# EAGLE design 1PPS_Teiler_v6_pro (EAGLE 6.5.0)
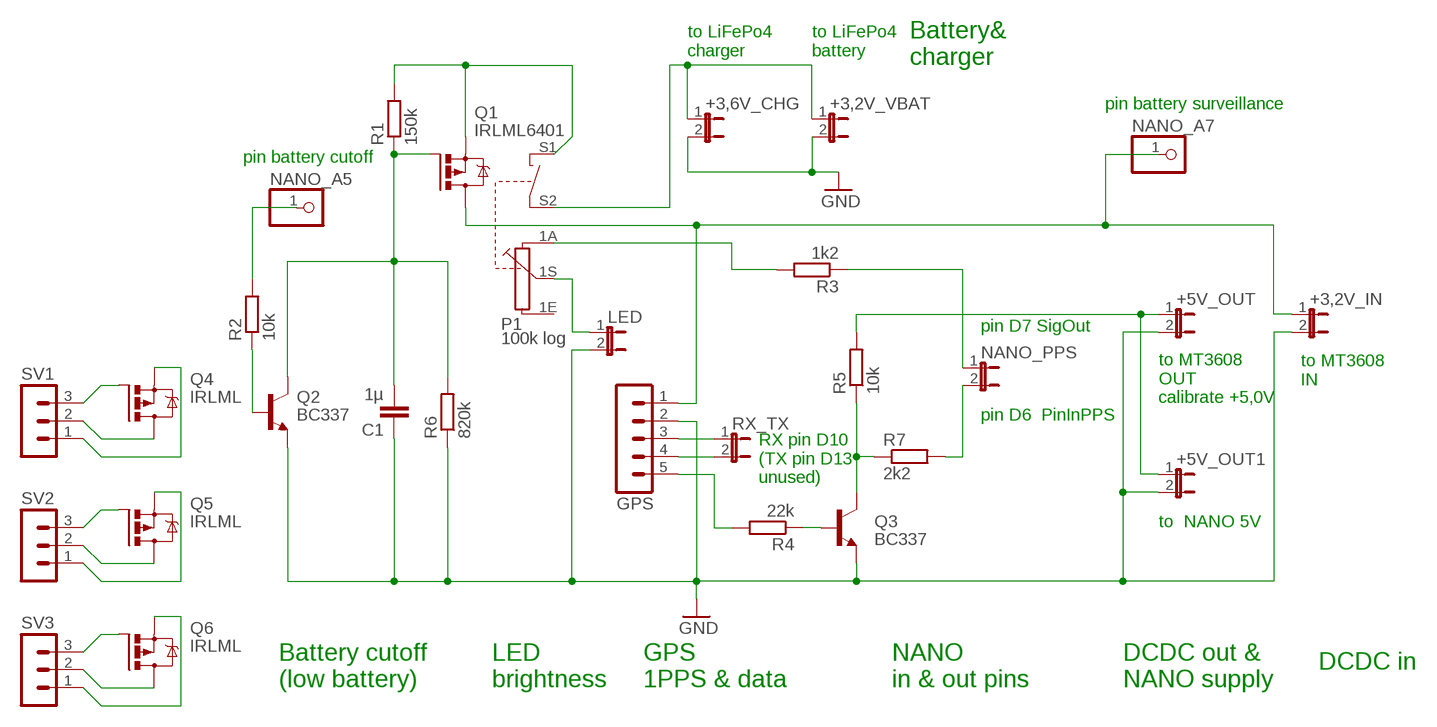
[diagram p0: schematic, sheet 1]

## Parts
+3,2V_IN  JP1E  [JP1]
+3,2V_VBAT  JP1E  [JP1]
+3,6V_CHG  JP1E  [JP1]
+5V_OUT  JP1E  [JP1]
+5V_OUT1  JP1E  [JP1]
C1  1µ  C-EU050-025X075  [C050-025X075]
GPS  MA05-1  [MA05-1]
LED  JP1E  [JP1]
NANO_A5  PINHD-1X1  [1X01]
NANO_A7  PINHD-1X1  [1X01]
NANO_PPS  JP1E  [JP1]
P1  100k log  PC16SV  [PC16SV]
Q1  IRLML6401  IRLML5203  [MICRO3]
Q2  BC337  BC337-40  [TO92]
Q3  BC337  2N4124-NPN-TO92-CBE  [TO92-CBE]
Q4  IRLML  IRLML5203  [MICRO3]
Q5  IRLML  IRLML5203  [MICRO3]
Q6  IRLML  IRLML5203  [MICRO3]
R1  150k  R-EU_0204/5  [0204/5]
R2  10k  R-EU_0204/5  [0204/5]
R3  1k2  R-EU_0204/7  [0204/7]
R4  22k  R-EU_0204/5  [0204/5]
R5  10k  R-EU_0204/7  [0204/7]
R6  820k  R-EU_0204/7  [0204/7]
R7  2k2  R-EU_0204/2V  [0204V]
RX_TX  JP1E  [JP1]
SV1  MA03-1  [MA03-1]
SV2  MA03-1  [MA03-1]
SV3  MA03-1  [MA03-1]

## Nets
3V2: +3,2V_IN.1 GPS.1 NANO_A7.1 Q1.3(D)
5V0: +5V_OUT1.1 +5V_OUT.1 R5.2
GND: +3,2V_IN.2 +3,2V_VBAT.2 +3,6V_CHG.2 +5V_OUT1.2 +5V_OUT.2 C1.1 GPS.2 LED.2 Q2.1(E) Q3.E R6.1
GPS_PPS: GPS.5 R4.2
LED+: LED.1 P1.1S
N$1: C1.2 Q1.1(G) Q2.3(C) R1.1 R6.2
N$2: NANO_A5.1 R2.2
N$3: Q3.B R4.1
N$4: P1.1A R3.2
N$5: Q4.1(G) SV1.3
N$6: Q2.2(B) R2.1
N$7: Q5.1(G) SV2.3
N$8: Q6.3(D) SV3.2
N$9: Q4.3(D) SV1.2
N$10: Q5.3(D) SV2.2
N$11: Q6.1(G) SV3.3
N$12: Q4.2(S) SV1.1
N$13: Q5.2(S) SV2.1
N$14: Q6.2(S) SV3.1
N$15: Q3.C R5.1 R7.1
NANO12_TO_LED: NANO_PPS.1 R3.1
PLUS: +3,2V_VBAT.1 +3,6V_CHG.1 P1.S2
PLUS_SWI: P1.S1 Q1.2(S) R1.2
PPS_IN_TO_NANO11: NANO_PPS.2 R7.2
RX: GPS.4 RX_TX.2
TX: GPS.3 RX_TX.1
Unconnected: P1.1E

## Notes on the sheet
- to LiFePo4
  charger
- to LiFePo4
  battery
- Battery&
  charger
- pin battery surveillance
- pin battery cutoff
- pin D7 SigOut
- to MT3608 
  IN
- to MT3608 
  OUT
  calibrate +5,0V
- pin D6  PinInPPS
- RX pin D10
  (TX pin D13
  unused)
- to  NANO 5V
- DCDC in
- Battery cutoff
  (low battery)
- LED
  brightness
- GPS 
  1PPS & data
- NANO
  in & out pins
- DCDC out &
  NANO supply

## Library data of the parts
+3,2V_IN +3,2V_VBAT +3,6V_CHG +5V_OUT +5V_OUT1 LED NANO_PPS RX_TX = jumper:JP1E: JUMPER
C1 = rcl:C-EU: CAPACITOR, European symbol
GPS = con-lstb:MA05-1: PIN HEADER; OC_FARNELL: unknown; OC_NEWARK: unknown
NANO_A5 NANO_A7 = pinhead:PINHD-1X1: PIN HEADER
P1 = piher:PC16SV: POTENTIOMETER vertical single carbon potentiometer with switch, 16 mm; OC_FARNELL: unknown; OC_NEWARK: unknown
Q1 Q4-Q6 = transistor-power:IRLML5203: HEXFET P-Channel Power MOSFET
Q2 = transistor-npn:BC337*: NPN Transistor
Q3 = transistor:*-NPN-: NPN Transistror BF959 corrected 2008.03.06
R1-R7 = resistor:R-EU_: RESISTOR, European symbol
SV1-SV3 = con-lstb:MA03-1: PIN HEADER; OC_FARNELL: unknown; OC_NEWARK: unknown

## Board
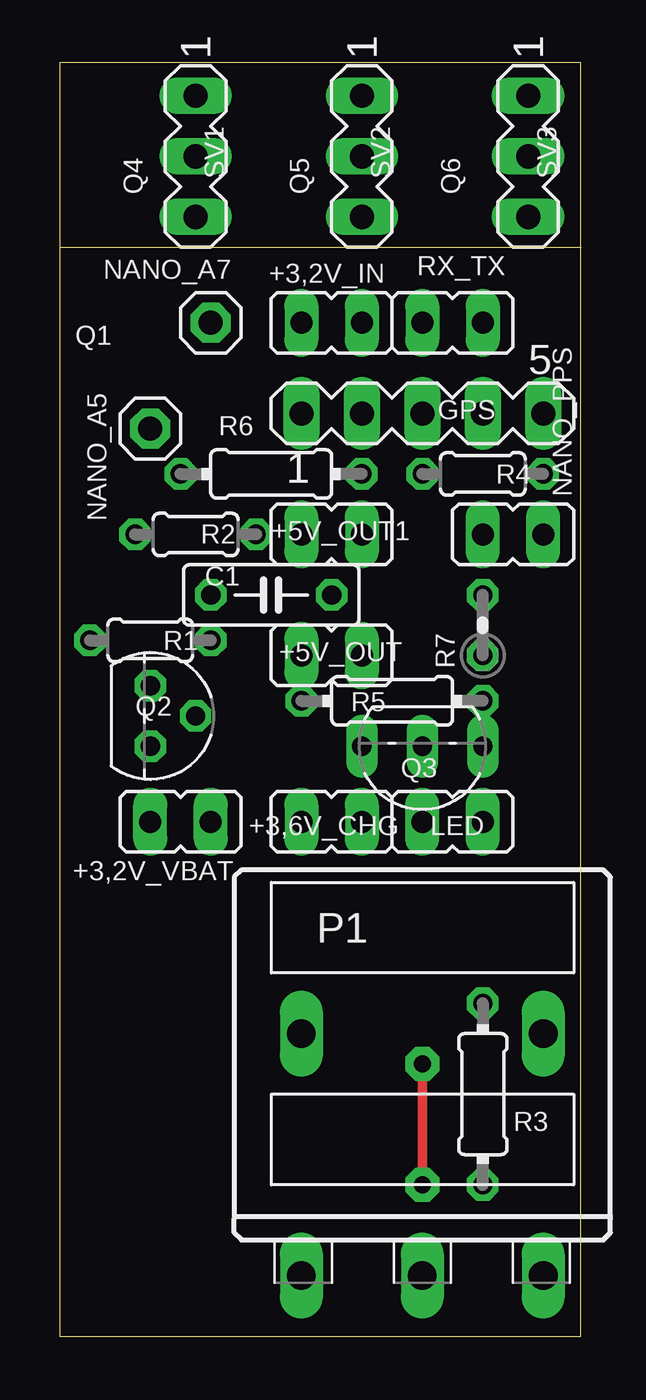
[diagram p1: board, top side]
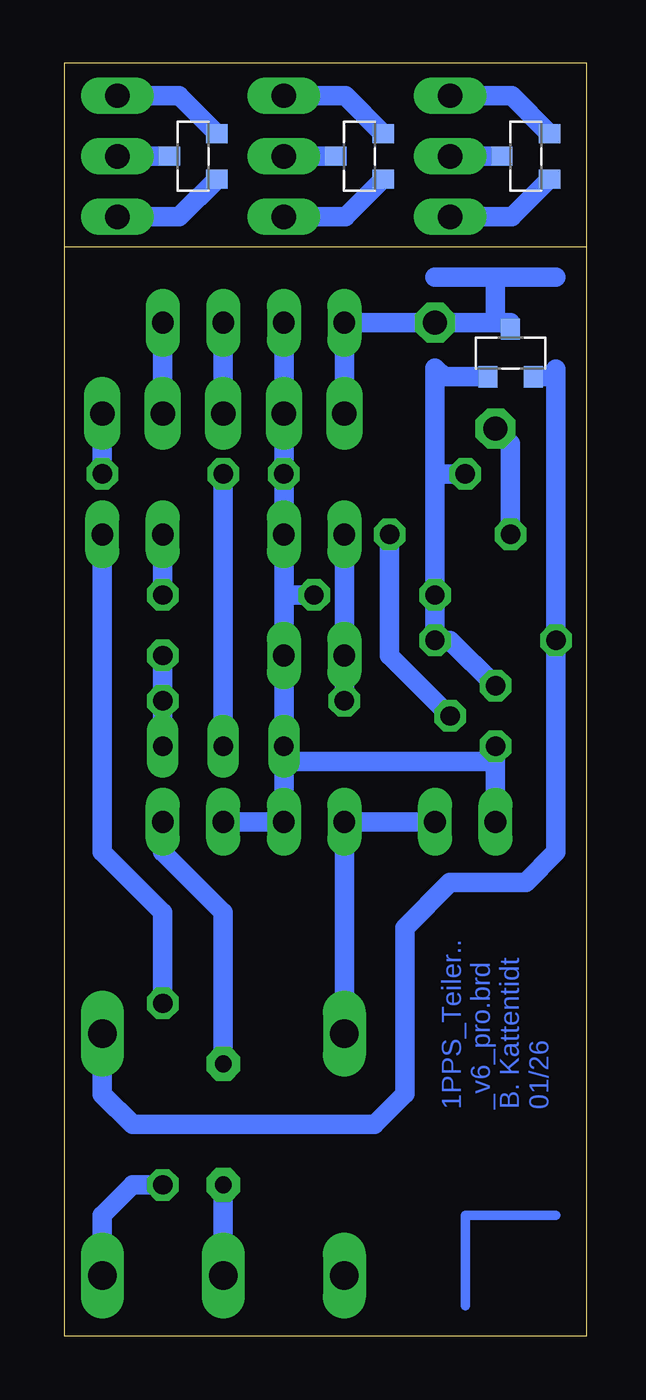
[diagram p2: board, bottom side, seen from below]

Size 21.91 x 53.46 mm. Coordinates in mm from the lower left corner, seen from the top.
Outline: 0,45.72 0,53.46 21.89,53.46 21.89,0 0,0 0,45.72
Outline: 0,45.72 21.91,45.72
Copper layers (1*16): Top 0.035mm / dielectric 1.5mm / Bottom 0.035mm
Design rules "default *": minimum track width 10mil, minimum drill 12mil, track to track 10mil, track to pad 10mil, pad to pad 10mil, via to via 10mil, smd to smd 8mil, copper to edge 20mil, drill to drill 8mil, minimum pad ring 10mil, minimum via ring 8mil, stop-mask expansion 4mil, vias tented up to drill 0mil, thermal gap 10mil

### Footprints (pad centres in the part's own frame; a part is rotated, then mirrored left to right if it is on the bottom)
JP1 = drill 0.914 long: 1 0,-1.27; 2 0,1.27
C050-025X075 = drill 0.813 octagon: 1 -2.54,0; 2 2.54,0
MA05-1 = drill 1.016 long: 1 -5.08,0; 2 -2.54,0; 3 0,0; 4 2.54,0; 5 5.08,0
1X01 = drill 1.016 pad 1.676 octagon: 1 0,0
PC16SV = drill 1.2 long: 1A -5.079,10.162; 1E 5.079,10.162; 1S 0,10.162; S1 -5.079,0.004; S2 5.079,0.004
MICRO3 = smd 0.8 x 0.9: 1 -0.95,-1; 2 0.95,-1; 3 0,1
TO92 = drill 0.813 octagon: 1 1.27,0; 2 0,1.905; 3 -1.27,0
TO92-CBE = drill 0.813 long: B 0,0; C -2.54,0; E 2.54,0
0204/5 = drill 0.813 octagon: 1 -2.54,0; 2 2.54,0
0204/7 = drill 0.813 octagon: 1 -3.81,0; 2 3.81,0
0204V = drill 0.813 octagon: 1 -1.27,0; 2 1.27,0
MA03-1 = drill 1.016 long: 1 -2.54,0; 2 0,0; 3 2.54,0

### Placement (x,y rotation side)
+3,2V_IN  11.43,42.55 270 top
+3,2V_VBAT  5.08,21.59 90 top
+3,6V_CHG  11.43,21.59 270 top
+5V_OUT  11.43,28.57 270 top
+5V_OUT1  11.43,33.66 270 top
C1  8.89,31.11 180 top
GPS  15.24,38.73 0 top
LED  16.51,21.59 90 top
NANO_A5  3.81,38.1 180 top
NANO_A7  6.35,42.55 0 top
NANO_PPS  19.05,33.66 90 top
P1  15.24,12.7 180 top
Q1  3.17,41.27 0 bottom
Q2  3.81,26.04 270 top
Q3  15.24,24.77 180 top
Q4  2.54,49.53 90 bottom
Q5  9.53,49.53 90 bottom
Q6  16.51,49.53 90 bottom
R1  3.81,29.21 180 top
R2  5.71,33.66 180 top
R3  17.78,10.16 270 top
R4  17.78,36.2 0 top
R5  13.97,26.67 180 top
R6  8.89,36.2 180 top
R7  17.78,29.84 90 top
RX_TX  16.51,42.55 270 top
SV1  5.71,49.53 270 top
SV2  12.7,49.53 270 top
SV3  19.68,49.53 270 top

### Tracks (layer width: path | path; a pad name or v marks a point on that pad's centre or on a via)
3V2
  Bottom 0.813: GPS.1 +3,2V_IN.1 NANO_A7.1 3.81,42.55 | 3.44,42.55 Q1.3 3.17,42.55 3.44,42.55 | 3.44,42.55 3.81,42.55 | 1.27,44.45 3.81,44.45 | 3.81,44.45 6.35,44.45 | 3.81,44.45 3.81,42.55
5V0
  Bottom 0.813: +5V_OUT1.1 +5V_OUT.1 R5.2
GND
  Bottom 0.813: LED.2 +3,6V_CHG.2 12.7,24.13 | +3,2V_IN.2 GPS.2 R6.1 +5V_OUT1.2 12.7,31.11 | Q2.1 3.81,24.13 | 3.81,24.13 12.7,24.13 | 12.7,24.13 Q3.E +5V_OUT.2 12.7,31.11 | +3,2V_VBAT.2 3.81,24.13 | C1.1 12.7,31.11
GPS_PPS
  Bottom 0.813: GPS.5 R4.2
LED+  (via drill 0.7 pad 1.42)
  Top 0.406: v15.24,6.35 v15.24,11.43
  Bottom 0.813: LED.1 17.78,20.32 15.24,17.78 v15.24,11.43 | v15.24,6.35 P1.1S
N$1
  Bottom 0.813: 6.35,36.2 6.35,40.64 5.99,40.27 Q1.1 | R6.2 6.35,36.2 | 6.35,36.2 C1.2 R1.1 5.71,29.21 Q2.3
N$2
  Bottom 0.813: R2.2 3.17,37.47 NANO_A5.1
N$3
  Bottom 0.813: R4.1 Q3.B
N$4
  Bottom 0.813: R3.2 19.05,6.35 20.32,5.08 P1.1A
N$5
  Bottom 0.813: SV1.3 3.13,46.99 Q4.1
N$6
  Bottom 0.813: Q2.2 8.26,28.57 R2.1
N$7
  Bottom 0.813: SV2.3 10.12,46.99 Q5.1
N$8
  Bottom 0.813: SV3.2 Q6.3
N$9
  Bottom 0.813: SV1.2 Q4.3
N$10
  Bottom 0.813: SV2.2 Q5.3
N$11
  Bottom 0.813: SV3.3 17.1,46.99 Q6.1
N$12
  Bottom 0.813: SV1.1 3.13,52.07 Q4.2
N$13
  Bottom 0.813: SV2.1 10.12,52.07 Q5.2
N$14
  Bottom 0.813: SV3.1 17.1,52.07 Q6.2
N$15
  Bottom 0.813: R7.1 R5.1 Q3.C
N$16
  Bottom 0.406: 1.27,5.08 5.08,5.08 5.08,1.27
NANO12_TO_LED
  Bottom 0.813: R3.1 17.78,17.78 20.32,20.32 NANO_PPS.1
PLUS
  Bottom 0.813: +3,2V_VBAT.1 +3,6V_CHG.1 P1.S2
PLUS_SWI
  Bottom 0.813: P1.S1 20.32,10.16 19.05,8.89 8.89,8.89 7.62,10.16 7.62,17.14 5.71,19.05 2.54,19.05 1.27,20.32 R1.2 1.27,40.27 | 1.27,40.59 1.27,40.27 | 1.27,40.27 Q1.2
PPS_IN_TO_NANO11
  Bottom 0.813: NANO_PPS.2 R7.2
RX
  Bottom 0.813: GPS.4 RX_TX.2
TX
  Bottom 0.813: GPS.3 RX_TX.1

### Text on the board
Bottom: 1PPS_Teiler.. / _v6_pro.brd / B. Kattentidt / 01/26
tValues: nano D6 / / nano D7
